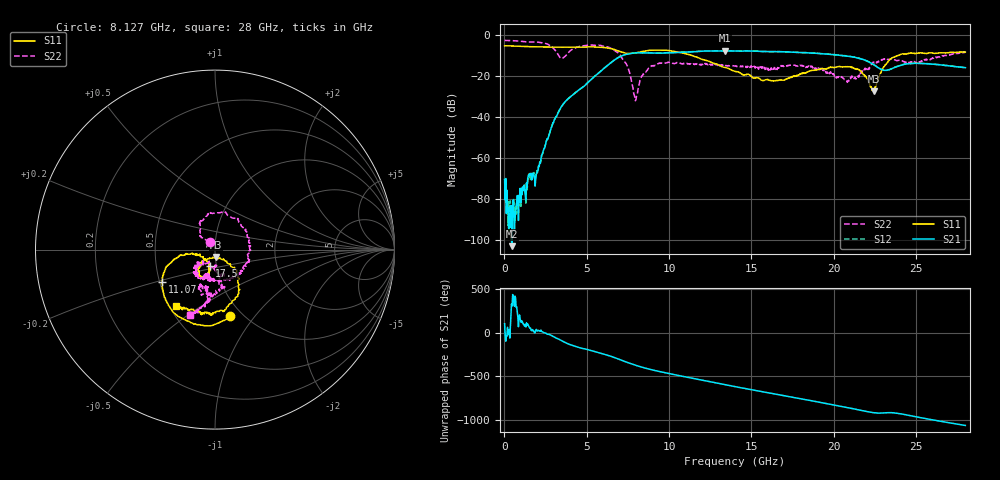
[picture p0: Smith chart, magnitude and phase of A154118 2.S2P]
!  2-Port S-parameters saved by WinCal
! VAR MeasName=S-Parameters (CALIBRATED_DATA) read from VNA (N5230A)
! VAR MeasDate=2015-9-10 14:34:37
! VAR NAME=A154118 2
! VAR FILENAME=A154118 2.S2P
! VAR DATE=2015-9-10 14:34:37
! VAR PHYS_PORTS=1,2
# Hz S DB R 50
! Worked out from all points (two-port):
!   801 points, 10 MHz to 28 GHz, reference 50 ohm
!   highest |S21| = -7.73 dB at 13.41 GHz (marker M1); lowest = -102.9 dB at 464.8 MHz (marker M2)
!   |S21| within 3 dB of the highest: 6.991 GHz to 21.19 GHz (14.2 GHz wide, 101 % of centre)
!   lowest |S11| = -27.5 dB at 22.44 GHz (marker M3), VSWR 1.09, Z = 50.5 - j4.23 ohm
!   |S11| at or under -10 dB: 11.38 GHz to 23.91 GHz (12.54 GHz wide, 71 % of centre)
!   |S22| runs from -32.0 to -2.7 dB; largest |S21 - S12| = 0.0079
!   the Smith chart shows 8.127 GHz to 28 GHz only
!   S11 on the Smith chart (normalised r, x): 8.127 GHz: 0.88, -0.76; 11.07 GHz: 0.52, -0.21; 17.5 GHz: 0.93, -0.17; 28 GHz: 0.54, -0.40
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1e7  -5.30 179.6  -70.40 102.4  -75.37 -169.5  -2.67 179.8
4.648375e8  -5.36 166.0  -102.94 -53.9  -85.86 160.5  -2.75 168.5
1.9693e9  -5.78 123.9  -66.96 20.1  -66.07 25.4  -3.48 129.1
2.66905e9  -5.88 102.5  -49.84 -20.2  -49.89 -19.3  -4.66 91.1
3.193862e9  -5.90 84.8  -39.07 -66.1  -39.05 -65.8  -8.71 25.6
3.753662e9  -5.92 64.8  -31.94 -119.5  -31.98 -119.1  -9.82 -108.8
4.698325e9  -6.00 27.8  -25.78 179.7  -25.78 179.9  -5.32 166.4
5.817925e9  -6.01 -19.0  -17.90 125.2  -17.84 125.5  -5.03 117.7
6.86755e9  -7.63 -60.0  -11.23 60.2  -11.15 60.0  -8.48 63.6
7.462338e9  -9.04 -69.6  -9.36 17.3  -9.30 17.2  -15.06 32.8
7.917175e9  -8.76 -73.5  -8.74 -12.2  -8.67 -12.2  -30.16 62.1
8.1271e9  -8.45 -76.8  -8.69 -25.0  -8.63 -25.2  -25.65 125.6
9.351662e9  -7.37 -107.8  -8.88 -84.7  -8.76 -84.9  -13.88 102.0
1.106605e10  -9.29 -148.7  -8.33 -151.8  -8.24 -152.6  -13.90 29.5
1.341021e10  -15.90 -172.0  -7.73 120.0  -7.73 119.3  -14.63 -66.8
1.4005e10  -17.69 -171.0  -7.82 98.5  -7.83 98.0  -15.17 -85.4
1.750375e10  -20.46 -108.0  -8.39 -23.7  -8.37 -24.0  -14.65 -119.6
1.869332e10  -17.25 -105.0  -8.80 -64.8  -8.82 -65.1  -15.30 -128.9
2.079258e10  -15.52 -119.7  -10.25 -140.4  -10.17 -140.9  -22.37 -112.9
2.243699e10  -27.47 -81.0  -14.54 158.8  -14.50 158.3  -13.24 -76.0
2.334666e10  -12.52 -55.4  -16.99 159.6  -16.93 159.0  -12.01 -100.0
2.8e10  -8.37 -124.8  -15.94 12.6  -15.98 11.6  -8.13 -111.1
